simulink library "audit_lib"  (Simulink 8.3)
settings: Solver=ode45  StartTime=0.0  StopTime=10.0  RelTol=1e-3
undefined symbols (not defined in the file or in its folder): convert, VerboseSignal
libraries: audit_lib x23, simulink x16

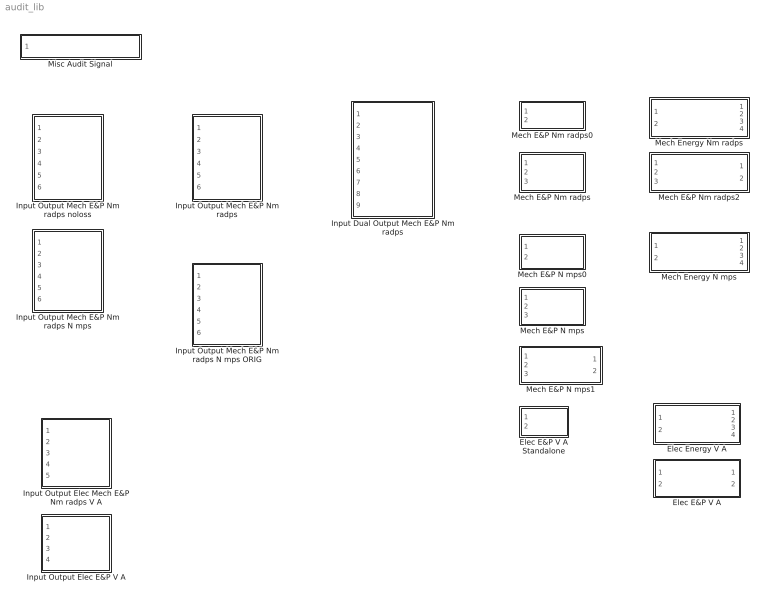
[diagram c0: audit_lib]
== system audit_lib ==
  Elec E&P V A : Subsystem
  Elec E&P V A Standalone : Subsystem
  Elec Energy V A : Subsystem  TreatAsAtomicUnit=on
  Input Dual Output Mech E&P Nm radps : Subsystem
  Input Output Elec E&P V A : Subsystem
  Input Output Elec Mech E&P Nm radps V A : Subsystem
  Input Output Mech E&P Nm radps : Subsystem
  Input Output Mech E&P Nm radps N mps : Subsystem
  Input Output Mech E&P Nm radps N mps ORIG : Subsystem
  Input Output Mech E&P Nm radps noloss : Subsystem
  Mech E&P N mps : Subsystem
  Mech E&P N mps0 : Subsystem
  Mech E&P N mps1 : Subsystem
  Mech E&P Nm radps : Subsystem
  Mech E&P Nm radps0 : Subsystem
  Mech E&P Nm radps2 : Subsystem
  Mech Energy N mps : Subsystem  TreatAsAtomicUnit=on
  Mech Energy Nm radps : Subsystem  TreatAsAtomicUnit=on
  Misc Audit Signal : Subsystem

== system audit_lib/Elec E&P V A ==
  volts_V : Inport
  curr_A : Inport  Port=2
  Compare To Constant : simulink/Logic and Bit Operations/Compare To Constant  relop=>=  const=1  OutDataTypeStr=boolean
  Constant : Constant  Value=VerboseSignal
  Subsystem : Subsystem
  pos_kJ : Outport
  neg_kJ : Outport  Port=2
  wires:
  volts_V/1 -> Subsystem/1(volts_V)
  curr_A/1 -> Subsystem/2(curr_A)
  Subsystem/1(pos_kJ) -> pos_kJ/1
  Subsystem/2(neg_kJ) -> neg_kJ/1
  Compare To Constant/1 -> Subsystem/Enable
  Constant/1 -> Compare To Constant/1

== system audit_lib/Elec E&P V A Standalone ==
  volts_V : Inport
  curr_A : Inport  Port=2
  Compare To Constant : simulink/Logic and Bit Operations/Compare To Constant  relop=>=  const=1  OutDataTypeStr=boolean
  Constant : Constant  Value=VerboseSignal
  Subsystem : Subsystem
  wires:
  volts_V/1 -> Subsystem/1(volts_V)
  curr_A/1 -> Subsystem/2(curr_A)
  Compare To Constant/1 -> Subsystem/Enable
  Constant/1 -> Compare To Constant/1

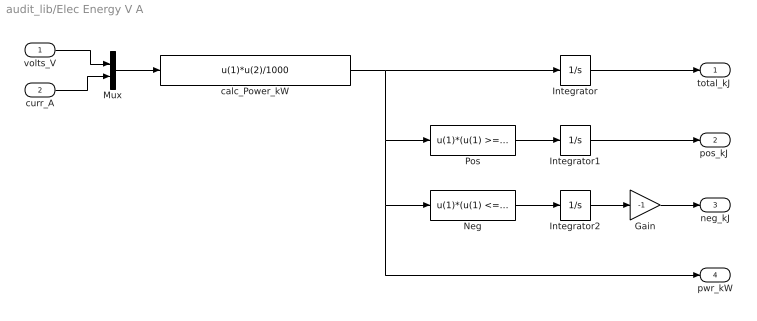
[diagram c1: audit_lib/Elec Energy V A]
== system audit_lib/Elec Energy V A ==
  volts_V : Inport
  curr_A : Inport  Port=2
  Gain : Gain  Gain=-1
  Integrator : Integrator  ZeroCross=off
  Integrator1 : Integrator  ZeroCross=off
  Integrator2 : Integrator  ZeroCross=off
  Mux : Mux  Inputs=2
  Neg : Fcn  Expr=u(1)*(u(1) <= 0)
  Pos : Fcn  Expr=u(1)*(u(1) >= 0)
  calc_Power_kW : Fcn  Expr=u(1)*u(2)/1000
  "total_kJ " : Outport
  "pos_kJ " : Outport  Port=2
  neg_kJ : Outport  Port=3
  pwr_kW : Outport  Port=4
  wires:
  calc_Power_kW/1 -> Pos/1, Neg/1, pwr_kW/1, Integrator/1
  Gain/1 -> neg_kJ/1
  Integrator1/1 -> "pos_kJ "/1
  Integrator2/1 -> Gain/1
  Neg/1 -> Integrator2/1
  Pos/1 -> Integrator1/1
  Integrator/1 -> "total_kJ "/1
  Mux/1 -> calc_Power_kW/1
  volts_V/1 -> Mux/1
  curr_A/1 -> Mux/2

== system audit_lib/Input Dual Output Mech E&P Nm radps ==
  trq_in_Nm : Inport
  spd_in_radps : Inport  Port=2
  iner_in_kgm2 : Inport  Port=3
  trq_out1_Nm : Inport  Port=4
  spd_out1_radps : Inport  Port=5
  iner_out1_kgm2 : Inport  Port=6
  trq_out2_Nm : Inport  Port=7
  spd_out2_radps : Inport  Port=8
  iner_out2_kgm : Inport  Port=9
  Compare To Constant : simulink/Logic and Bit Operations/Compare To Constant  relop=>=  const=1  OutDataTypeStr=boolean
  Constant : Constant  Value=VerboseSignal
  Subsystem : Subsystem
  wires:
  trq_in_Nm/1 -> Subsystem/1(trq_in_Nm)
  spd_in_radps/1 -> Subsystem/2(spd_in_radps)
  iner_in_kgm2/1 -> Subsystem/3(iner_in_kgm2)
  trq_out1_Nm/1 -> Subsystem/4(trq_out1_Nm)
  spd_out1_radps/1 -> Subsystem/5(spd_out1_radps)
  iner_out1_kgm2/1 -> Subsystem/6(iner_out1_kgm2)
  trq_out2_Nm/1 -> Subsystem/7(trq_out2_Nm)
  spd_out2_radps/1 -> Subsystem/8(spd_out2_radps)
  iner_out2_kgm/1 -> Subsystem/9(iner_out2_kgm)
  Compare To Constant/1 -> Subsystem/Enable
  Constant/1 -> Compare To Constant/1

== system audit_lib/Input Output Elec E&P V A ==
  volts_in_V : Inport
  curr_in_A : Inport  Port=2
  volts_out_V : Inport  Port=3
  curr_out_A : Inport  Port=4
  Compare To Constant : simulink/Logic and Bit Operations/Compare To Constant  relop=>=  const=1  OutDataTypeStr=boolean
  Constant : Constant  Value=VerboseSignal
  Subsystem : Subsystem
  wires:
  volts_in_V/1 -> Subsystem/1(volts_in_V)
  curr_in_A/1 -> Subsystem/2(curr_in_A)
  volts_out_V/1 -> Subsystem/3(volts_out_V)
  curr_out_A/1 -> Subsystem/4(curr_out_A)
  Compare To Constant/1 -> Subsystem/Enable
  Constant/1 -> Compare To Constant/1

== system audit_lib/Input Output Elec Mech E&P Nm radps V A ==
  volts_in_V : Inport
  curr_in_A : Inport  Port=2
  trq_out_Nm : Inport  Port=3
  spd_out_radps : Inport  Port=4
  iner_out_kgm2 : Inport  Port=5
  Compare To Constant : simulink/Logic and Bit Operations/Compare To Constant  relop=>=  const=1  OutDataTypeStr=boolean
  Constant : Constant  Value=VerboseSignal
  Subsystem : Subsystem
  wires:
  volts_in_V/1 -> Subsystem/1(volts_in_V)
  curr_in_A/1 -> Subsystem/2(curr_in_A)
  trq_out_Nm/1 -> Subsystem/3(trq_out_Nm)
  spd_out_radps/1 -> Subsystem/4(spd_out_radps)
  iner_out_kgm2/1 -> Subsystem/5(iner_out_kgm2)
  Compare To Constant/1 -> Subsystem/Enable
  Constant/1 -> Compare To Constant/1

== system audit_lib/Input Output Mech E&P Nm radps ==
  trq_in_Nm : Inport
  spd_in_radps : Inport  Port=2
  iner_in_kgm2 : Inport  Port=3
  trq_out_Nm : Inport  Port=4
  spd_out_radps : Inport  Port=5
  iner_out_kgm2 : Inport  Port=6
  Compare To Constant : simulink/Logic and Bit Operations/Compare To Constant  relop=>=  const=1  OutDataTypeStr=boolean
  Constant : Constant  Value=VerboseSignal
  Subsystem : Subsystem
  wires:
  trq_in_Nm/1 -> Subsystem/1(trq_in_Nm)
  spd_in_radps/1 -> Subsystem/2(spd_in_radps)
  iner_in_kgm2/1 -> Subsystem/3(iner_in_kgm2)
  trq_out_Nm/1 -> Subsystem/4(trq_out_Nm)
  spd_out_radps/1 -> Subsystem/5(spd_out_radps)
  iner_out_kgm2/1 -> Subsystem/6(iner_out_kgm2)
  Compare To Constant/1 -> Subsystem/Enable
  Constant/1 -> Compare To Constant/1

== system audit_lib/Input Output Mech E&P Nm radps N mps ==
  trq_in_Nm : Inport
  spd_in_radps : Inport  Port=2
  iner_in_kgm2 : Inport  Port=3
  frc_out_N : Inport  Port=4
  spd_out_mps : Inport  Port=5
  mass_out_kg : Inport  Port=6
  Compare To Constant : simulink/Logic and Bit Operations/Compare To Constant  relop=>=  const=1  OutDataTypeStr=boolean
  Constant : Constant  Value=VerboseSignal
  Subsystem : Subsystem
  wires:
  trq_in_Nm/1 -> Subsystem/1(trq_in_Nm)
  spd_in_radps/1 -> Subsystem/2(spd_in_radps)
  iner_in_kgm2/1 -> Subsystem/3(iner_in_kgm2)
  frc_out_N/1 -> Subsystem/4(frc_out_N)
  spd_out_mps/1 -> Subsystem/5(spd_out_mps)
  mass_out_kg/1 -> Subsystem/6(mass_out_kg)
  Compare To Constant/1 -> Subsystem/Enable
  Constant/1 -> Compare To Constant/1

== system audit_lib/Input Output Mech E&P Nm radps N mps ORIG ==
  trq_in_Nm : Inport
  spd_in_radps : Inport  Port=2
  iner_in_kgm2 : Inport  Port=3
  frc_out_N : Inport  Port=4
  spd_out_mps : Inport  Port=5
  mass_out_kg : Inport  Port=6
  Compare To Constant : simulink/Logic and Bit Operations/Compare To Constant  relop=>=  const=1  OutDataTypeStr=boolean
  Constant : Constant  Value=VerboseSignal
  Subsystem : Subsystem
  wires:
  Constant/1 -> Compare To Constant/1
  Compare To Constant/1 -> Subsystem/Enable
  mass_out_kg/1 -> Subsystem/6(mass_out_kg)
  spd_out_mps/1 -> Subsystem/5(spd_out_mps)
  frc_out_N/1 -> Subsystem/4(frc_out_N)
  iner_in_kgm2/1 -> Subsystem/3(iner_in_kgm2)
  spd_in_radps/1 -> Subsystem/2(spd_in_radps)
  trq_in_Nm/1 -> Subsystem/1(trq_in_Nm)

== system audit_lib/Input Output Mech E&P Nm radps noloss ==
  trq_in_Nm : Inport
  spd_in_radps : Inport  Port=2
  iner_in_kgm2 : Inport  Port=3
  trq_out_Nm : Inport  Port=4
  spd_out_radps : Inport  Port=5
  iner_out_kgm2 : Inport  Port=6
  Compare To Constant : simulink/Logic and Bit Operations/Compare To Constant  relop=>=  const=1  OutDataTypeStr=boolean
  Constant : Constant  Value=VerboseSignal
  Subsystem : Subsystem
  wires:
  trq_in_Nm/1 -> Subsystem/1(trq_in_Nm)
  spd_in_radps/1 -> Subsystem/2(spd_in_radps)
  iner_in_kgm2/1 -> Subsystem/3(iner_in_kgm2)
  trq_out_Nm/1 -> Subsystem/4(trq_out_Nm)
  spd_out_radps/1 -> Subsystem/5(spd_out_radps)
  iner_out_kgm2/1 -> Subsystem/6(iner_out_kgm2)
  Compare To Constant/1 -> Subsystem/Enable
  Constant/1 -> Compare To Constant/1

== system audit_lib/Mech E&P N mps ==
  force_N : Inport
  spd_mps : Inport  Port=2
  mass_kg : Inport  Port=3
  Compare To Constant : simulink/Logic and Bit Operations/Compare To Constant  relop=>=  const=1  OutDataTypeStr=boolean
  Constant : Constant  Value=VerboseSignal
  Subsystem : Subsystem
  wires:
  force_N/1 -> Subsystem/1(force_N)
  spd_mps/1 -> Subsystem/2(spd_mps)
  mass_kg/1 -> Subsystem/3(mass_kg)
  Compare To Constant/1 -> Subsystem/Enable
  Constant/1 -> Compare To Constant/1

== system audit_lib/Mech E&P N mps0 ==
  force_N : Inport
  spd_mps : Inport  Port=2
  Compare To Constant : simulink/Logic and Bit Operations/Compare To Constant  relop=>=  const=1  OutDataTypeStr=boolean
  Constant : Constant  Value=VerboseSignal
  Subsystem : Subsystem
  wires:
  force_N/1 -> Subsystem/1(force_N)
  spd_mps/1 -> Subsystem/2(spd_mps)
  Compare To Constant/1 -> Subsystem/Enable
  Constant/1 -> Compare To Constant/1

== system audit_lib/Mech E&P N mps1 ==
  force_N : Inport
  spd_mps : Inport  Port=2
  mass_kg : Inport  Port=3
  Compare To Constant : simulink/Logic and Bit Operations/Compare To Constant  relop=>=  const=1  OutDataTypeStr=boolean
  Constant : Constant  Value=VerboseSignal
  Subsystem : Subsystem
  pos_kJ : Outport
  neg_kJ : Outport  Port=2
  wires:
  Constant/1 -> Compare To Constant/1
  Compare To Constant/1 -> Subsystem/Enable
  mass_kg/1 -> Subsystem/3(mass_kg)
  spd_mps/1 -> Subsystem/2(spd_mps)
  force_N/1 -> Subsystem/1(force_N)
  Subsystem/1(pos_kJ) -> pos_kJ/1
  Subsystem/2(neg_kJ) -> neg_kJ/1

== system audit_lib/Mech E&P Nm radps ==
  " trq_Nm" : Inport
  spd_radps : Inport  Port=2
  iner_kgm2 : Inport  Port=3
  Compare To Constant : simulink/Logic and Bit Operations/Compare To Constant  relop=>=  const=1  OutDataTypeStr=boolean
  Constant : Constant  Value=VerboseSignal
  Subsystem : Subsystem
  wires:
  " trq_Nm"/1 -> Subsystem/1(" trq_Nm")
  spd_radps/1 -> Subsystem/2(spd_radps)
  iner_kgm2/1 -> Subsystem/3(iner_kgm2)
  Compare To Constant/1 -> Subsystem/Enable
  Constant/1 -> Compare To Constant/1

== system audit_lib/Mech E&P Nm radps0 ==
  trq_Nm : Inport
  spd_radps : Inport  Port=2
  Compare To Constant : simulink/Logic and Bit Operations/Compare To Constant  relop=>=  const=1  OutDataTypeStr=boolean
  Constant : Constant  Value=VerboseSignal
  Subsystem : Subsystem
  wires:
  trq_Nm/1 -> Subsystem/1(trq_Nm)
  spd_radps/1 -> Subsystem/2(spd_radps)
  Compare To Constant/1 -> Subsystem/Enable
  Constant/1 -> Compare To Constant/1

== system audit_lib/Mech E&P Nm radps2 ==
  " trq_Nm" : Inport
  spd_radps : Inport  Port=2
  iner_kgm2 : Inport  Port=3
  Compare To Constant : simulink/Logic and Bit Operations/Compare To Constant  relop=>=  const=1  OutDataTypeStr=boolean
  Constant : Constant  Value=VerboseSignal
  Subsystem : Subsystem
  pos_kJ : Outport
  neg_kJ : Outport  Port=2
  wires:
  " trq_Nm"/1 -> Subsystem/1(" trq_Nm")
  spd_radps/1 -> Subsystem/2(spd_radps)
  iner_kgm2/1 -> Subsystem/3(iner_kgm2)
  Compare To Constant/1 -> Subsystem/Enable
  Subsystem/1(pos_kJ) -> pos_kJ/1
  Subsystem/2(neg_kJ) -> neg_kJ/1
  Constant/1 -> Compare To Constant/1

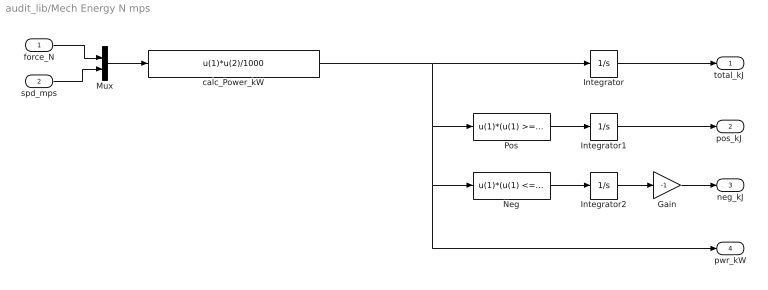
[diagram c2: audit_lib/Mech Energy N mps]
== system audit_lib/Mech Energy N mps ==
  force_N : Inport
  spd_mps : Inport  Port=2
  Gain : Gain  Gain=-1
  Integrator : Integrator  ZeroCross=off
  Integrator1 : Integrator  ZeroCross=off
  Integrator2 : Integrator  ZeroCross=off
  Mux : Mux  Inputs=2
  Neg : Fcn  Expr=u(1)*(u(1) <= 0)
  Pos : Fcn  Expr=u(1)*(u(1) >= 0)
  calc_Power_kW : Fcn  Expr=u(1)*u(2)/1000
  "total_kJ " : Outport
  "pos_kJ " : Outport  Port=2
  neg_kJ : Outport  Port=3
  pwr_kW : Outport  Port=4
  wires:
  spd_mps/1 -> Mux/2
  force_N/1 -> Mux/1
  Mux/1 -> calc_Power_kW/1
  Integrator/1 -> "total_kJ "/1
  Pos/1 -> Integrator1/1
  Neg/1 -> Integrator2/1
  Integrator2/1 -> Gain/1
  Integrator1/1 -> "pos_kJ "/1
  Gain/1 -> neg_kJ/1
  calc_Power_kW/1 -> Integrator/1, pwr_kW/1, Neg/1, Pos/1

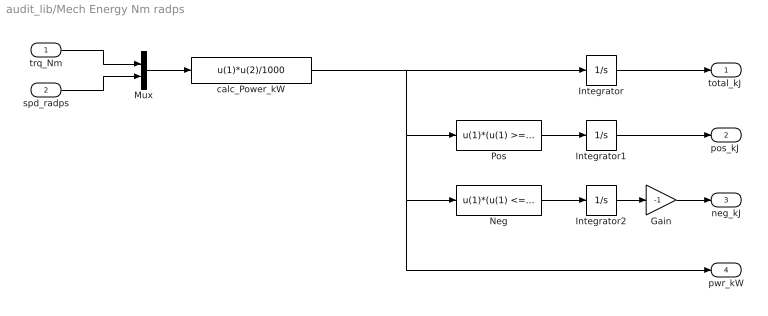
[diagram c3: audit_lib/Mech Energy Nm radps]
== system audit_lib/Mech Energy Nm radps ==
  trq_Nm : Inport
  spd_radps : Inport  Port=2
  Gain : Gain  Gain=-1
  Integrator : Integrator  ZeroCross=off
  Integrator1 : Integrator  ZeroCross=off
  Integrator2 : Integrator  ZeroCross=off
  Mux : Mux  Inputs=2
  Neg : Fcn  Expr=u(1)*(u(1) <= 0)
  Pos : Fcn  Expr=u(1)*(u(1) >= 0)
  calc_Power_kW : Fcn  Expr=u(1)*u(2)/1000
  "total_kJ " : Outport
  "pos_kJ " : Outport  Port=2
  neg_kJ : Outport  Port=3
  pwr_kW : Outport  Port=4
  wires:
  Integrator/1 -> "total_kJ "/1
  Mux/1 -> calc_Power_kW/1
  trq_Nm/1 -> Mux/1
  spd_radps/1 -> Mux/2
  Pos/1 -> Integrator1/1
  Neg/1 -> Integrator2/1
  Integrator2/1 -> Gain/1
  Integrator1/1 -> "pos_kJ "/1
  Gain/1 -> neg_kJ/1
  calc_Power_kW/1 -> Integrator/1, pwr_kW/1, Neg/1, Pos/1

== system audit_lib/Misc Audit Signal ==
  Var : Inport
  Compare To Constant : simulink/Logic and Bit Operations/Compare To Constant  relop=>=  const=1  OutDataTypeStr=boolean
  Constant : Constant  Value=VerboseSignal
  Subsystem : Subsystem
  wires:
  Var/1 -> Subsystem/1(In1)
  Compare To Constant/1 -> Subsystem/Enable
  Constant/1 -> Compare To Constant/1

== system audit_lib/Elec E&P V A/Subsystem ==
  volts_V : Inport
  curr_A : Inport  Port=2
  Enable : EnablePort  ZeroCross=off
  Elec Energy V A : audit_lib/Elec Energy V A
  amps_to_workspace : ToWorkspace  VariableName=audit__elec__emachine_Amps  SampleTime=-1
  energy_to_workspace : ToWorkspace  VariableName=audit__elec__emachine_kJ  SampleTime=-1
  neg_energy_to_workspace : ToWorkspace  VariableName=audit__elec__emachine_neg_kJ  SampleTime=-1
  pos_energy_to_workspace : ToWorkspace  VariableName=audit__elec__emachine_pos_kJ  SampleTime=-1
  power_to_workspace : ToWorkspace  VariableName=audit__elec__emachine_kW  SampleTime=-1
  volts_to_workspace : ToWorkspace  VariableName=audit__elec__emachine_Volts  SampleTime=-1
  pos_kJ : Outport  InitialOutput=0
  neg_kJ : Outport  Port=2  InitialOutput=0
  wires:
  Elec Energy V A/3 -> neg_kJ/1, neg_energy_to_workspace/1
  Elec Energy V A/4 -> power_to_workspace/1
  Elec Energy V A/2 -> pos_kJ/1, pos_energy_to_workspace/1
  Elec Energy V A/1 -> energy_to_workspace/1
  volts_V/1 -> volts_to_workspace/1, Elec Energy V A/1
  curr_A/1 -> amps_to_workspace/1, Elec Energy V A/2

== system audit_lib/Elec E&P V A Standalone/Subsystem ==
  volts_V : Inport
  curr_A : Inport  Port=2
  Enable : EnablePort  ZeroCross=off
  Elec Energy V A : audit_lib/Elec Energy V A
  amps_to_workspace : ToWorkspace  VariableName=audit__elec__emachine_Amps  SampleTime=-1
  energy_to_workspace : ToWorkspace  VariableName=audit__elec__emachine_kJ  SampleTime=-1
  neg_energy_to_workspace : ToWorkspace  VariableName=audit__elec__emachine_neg_kJ  SampleTime=-1
  pos_energy_to_workspace : ToWorkspace  VariableName=audit__elec__emachine_pos_kJ  SampleTime=-1
  power_to_workspace : ToWorkspace  VariableName=audit__elec__emachine_kW  SampleTime=-1
  volts_to_workspace : ToWorkspace  VariableName=audit__elec__emachine_Volts  SampleTime=-1
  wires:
  volts_V/1 -> Elec Energy V A/1, volts_to_workspace/1
  curr_A/1 -> Elec Energy V A/2, amps_to_workspace/1
  Elec Energy V A/3 -> neg_energy_to_workspace/1
  Elec Energy V A/2 -> pos_energy_to_workspace/1
  Elec Energy V A/4 -> power_to_workspace/1
  Elec Energy V A/1 -> energy_to_workspace/1

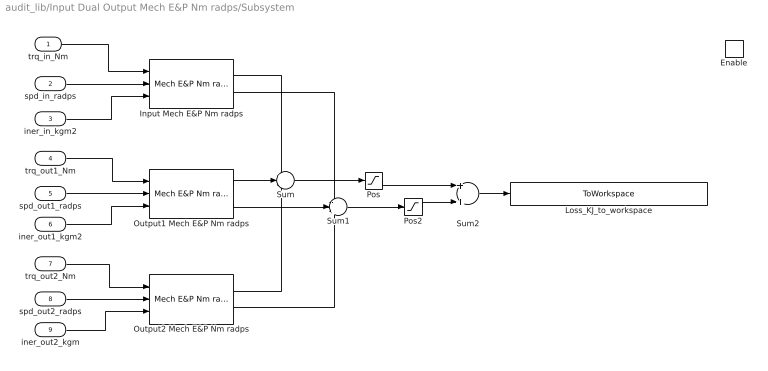
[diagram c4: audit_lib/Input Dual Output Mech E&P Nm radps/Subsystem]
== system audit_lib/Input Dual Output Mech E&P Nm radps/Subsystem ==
  trq_in_Nm : Inport
  spd_in_radps : Inport  Port=2
  iner_in_kgm2 : Inport  Port=3
  trq_out1_Nm : Inport  Port=4
  spd_out1_radps : Inport  Port=5
  iner_out1_kgm2 : Inport  Port=6
  trq_out2_Nm : Inport  Port=7
  spd_out2_radps : Inport  Port=8
  iner_out2_kgm : Inport  Port=9
  Enable : EnablePort  ZeroCross=off
  Input Mech E&P Nm radps : audit_lib/Mech E&P Nm radps2  base_name=clutch__input  VerboseSignal=REVS.verbose
  Loss_KJ_to_workspace : ToWorkspace  VariableName=audit__mech__clutch__loss_kJ  SampleTime=-1
  Output1 Mech E&P Nm radps : audit_lib/Mech E&P Nm radps2  base_name=clutch__output1  VerboseSignal=REVS.verbose
  Output2 Mech E&P Nm radps : audit_lib/Mech E&P Nm radps2  base_name=clutch__output2  VerboseSignal=REVS.verbose
  Pos : Saturate  UpperLimit=Inf  LowerLimit=0  ZeroCross=off
  Pos2 : Saturate  UpperLimit=Inf  LowerLimit=0  ZeroCross=off
  Sum : Sum  Inputs=+--
  Sum1 : Sum  Inputs=-++
  Sum2 : Sum
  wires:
  Output2 Mech E&P Nm radps/1 -> Sum/3
  Output2 Mech E&P Nm radps/2 -> Sum1/3
  iner_out2_kgm/1 -> Output2 Mech E&P Nm radps/3
  spd_out2_radps/1 -> Output2 Mech E&P Nm radps/2
  trq_out2_Nm/1 -> Output2 Mech E&P Nm radps/1
  Pos2/1 -> Sum2/2
  Pos/1 -> Sum2/1
  trq_in_Nm/1 -> Input Mech E&P Nm radps/1
  spd_in_radps/1 -> Input Mech E&P Nm radps/2
  trq_out1_Nm/1 -> Output1 Mech E&P Nm radps/1
  spd_out1_radps/1 -> Output1 Mech E&P Nm radps/2
  iner_in_kgm2/1 -> Input Mech E&P Nm radps/3
  iner_out1_kgm2/1 -> Output1 Mech E&P Nm radps/3
  Input Mech E&P Nm radps/1 -> Sum/1
  Output1 Mech E&P Nm radps/1 -> Sum/2
  Output1 Mech E&P Nm radps/2 -> Sum1/2
  Input Mech E&P Nm radps/2 -> Sum1/1
  Sum/1 -> Pos/1
  Sum1/1 -> Pos2/1
  Sum2/1 -> Loss_KJ_to_workspace/1

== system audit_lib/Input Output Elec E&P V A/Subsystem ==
  volts_in_V : Inport
  curr_in_A : Inport  Port=2
  volts_out_V : Inport  Port=3
  curr_out_A : Inport  Port=4
  Enable : EnablePort
  Input Elec E&P V A : audit_lib/Elec E&P V A  base_name=econverter__input  VerboseSignal=REVS.verbose
  Loss_KJ_to_workspace : ToWorkspace  VariableName=audit__elec__econverter__loss_kJ  SampleTime=-1
  Output Elec E&P V A : audit_lib/Elec E&P V A  base_name=econverter__output  VerboseSignal=REVS.verbose
  Pos : Saturate  UpperLimit=Inf  LowerLimit=0  ZeroCross=off
  Pos2 : Saturate  UpperLimit=Inf  LowerLimit=0  ZeroCross=off
  Sum : Sum  Inputs=+-|
  Sum1 : Sum  Inputs=|-+
  Sum2 : Sum
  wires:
  Input Elec E&P V A/1 -> Sum/1
  Sum2/1 -> Loss_KJ_to_workspace/1
  Sum1/1 -> Pos2/1
  Sum/1 -> Pos/1
  Output Elec E&P V A/2 -> Sum1/2
  Input Elec E&P V A/2 -> Sum1/1
  Output Elec E&P V A/1 -> Sum/2
  curr_in_A/1 -> Input Elec E&P V A/2
  volts_in_V/1 -> Input Elec E&P V A/1
  Pos/1 -> Sum2/2
  Pos2/1 -> Sum2/1
  curr_out_A/1 -> Output Elec E&P V A/2
  volts_out_V/1 -> Output Elec E&P V A/1

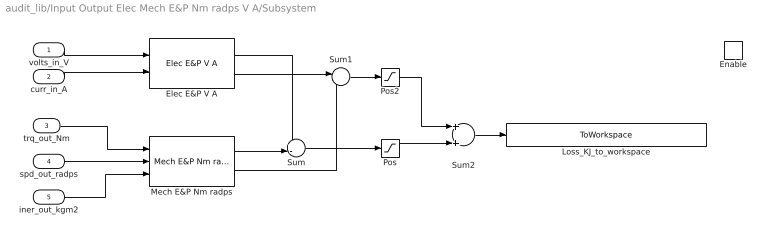
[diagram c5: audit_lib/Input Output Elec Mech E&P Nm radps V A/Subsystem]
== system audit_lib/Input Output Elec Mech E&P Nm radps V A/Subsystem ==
  volts_in_V : Inport
  curr_in_A : Inport  Port=2
  trq_out_Nm : Inport  Port=3
  spd_out_radps : Inport  Port=4
  iner_out_kgm2 : Inport  Port=5
  Enable : EnablePort
  Elec E&P V A : audit_lib/Elec E&P V A  base_name=emachine__input  VerboseSignal=REVS.verbose
  Loss_KJ_to_workspace : ToWorkspace  VariableName=audit__mech__emachine__loss_kJ  SampleTime=-1
  Mech E&P Nm radps : audit_lib/Mech E&P Nm radps2  base_name=emachine__output  VerboseSignal=REVS.verbose
  Pos : Saturate  UpperLimit=Inf  LowerLimit=0  ZeroCross=off
  Pos2 : Saturate  UpperLimit=Inf  LowerLimit=0  ZeroCross=off
  Sum : Sum  Inputs=+-|
  Sum1 : Sum  Inputs=|-+
  Sum2 : Sum
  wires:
  Pos2/1 -> Sum2/1
  Pos/1 -> Sum2/2
  trq_out_Nm/1 -> Mech E&P Nm radps/1
  spd_out_radps/1 -> Mech E&P Nm radps/2
  volts_in_V/1 -> Elec E&P V A/1
  curr_in_A/1 -> Elec E&P V A/2
  iner_out_kgm2/1 -> Mech E&P Nm radps/3
  Mech E&P Nm radps/1 -> Sum/2
  Elec E&P V A/2 -> Sum1/1
  Mech E&P Nm radps/2 -> Sum1/2
  Sum/1 -> Pos/1
  Sum1/1 -> Pos2/1
  Sum2/1 -> Loss_KJ_to_workspace/1
  Elec E&P V A/1 -> Sum/1

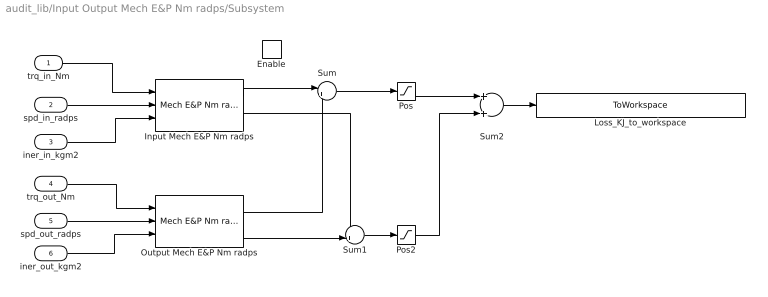
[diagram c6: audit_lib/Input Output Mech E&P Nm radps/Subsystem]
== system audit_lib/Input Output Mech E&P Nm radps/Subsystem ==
  trq_in_Nm : Inport
  spd_in_radps : Inport  Port=2
  iner_in_kgm2 : Inport  Port=3
  trq_out_Nm : Inport  Port=4
  spd_out_radps : Inport  Port=5
  iner_out_kgm2 : Inport  Port=6
  Enable : EnablePort  ZeroCross=off
  Input Mech E&P Nm radps : audit_lib/Mech E&P Nm radps2  base_name=torque_converter__input  VerboseSignal=REVS.verbose
  Loss_KJ_to_workspace : ToWorkspace  VariableName=audit__mech__torque_converter__loss_kJ  SampleTime=-1
  Output Mech E&P Nm radps : audit_lib/Mech E&P Nm radps2  base_name=torque_converter__output  VerboseSignal=REVS.verbose
  Pos : Saturate  UpperLimit=Inf  LowerLimit=0  ZeroCross=off
  Pos2 : Saturate  UpperLimit=Inf  LowerLimit=0  ZeroCross=off
  Sum : Sum  Inputs=|+-
  Sum1 : Sum  Inputs=-+|
  Sum2 : Sum
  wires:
  Pos2/1 -> Sum2/2
  Pos/1 -> Sum2/1
  trq_in_Nm/1 -> Input Mech E&P Nm radps/1
  spd_in_radps/1 -> Input Mech E&P Nm radps/2
  trq_out_Nm/1 -> Output Mech E&P Nm radps/1
  spd_out_radps/1 -> Output Mech E&P Nm radps/2
  iner_in_kgm2/1 -> Input Mech E&P Nm radps/3
  iner_out_kgm2/1 -> Output Mech E&P Nm radps/3
  Input Mech E&P Nm radps/1 -> Sum/1
  Output Mech E&P Nm radps/1 -> Sum/2
  Output Mech E&P Nm radps/2 -> Sum1/2
  Input Mech E&P Nm radps/2 -> Sum1/1
  Sum/1 -> Pos/1
  Sum1/1 -> Pos2/1
  Sum2/1 -> Loss_KJ_to_workspace/1

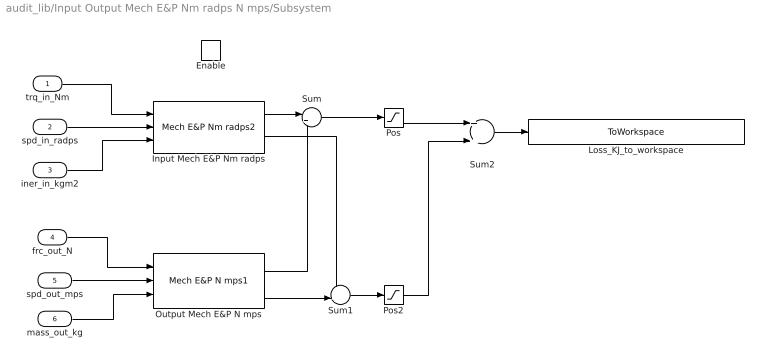
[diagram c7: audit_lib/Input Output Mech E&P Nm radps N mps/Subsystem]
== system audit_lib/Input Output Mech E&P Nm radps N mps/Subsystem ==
  trq_in_Nm : Inport
  spd_in_radps : Inport  Port=2
  iner_in_kgm2 : Inport  Port=3
  frc_out_N : Inport  Port=4
  spd_out_mps : Inport  Port=5
  mass_out_kg : Inport  Port=6
  Enable : EnablePort  ZeroCross=off
  Input Mech E&P Nm radps : audit_lib/Mech E&P Nm radps2  base_name=device__input  VerboseSignal=REVS.verbose
  Loss_KJ_to_workspace : ToWorkspace  VariableName=audit__mech__device__loss_kJ  SampleTime=-1
  Output Mech E&P N mps : audit_lib/Mech E&P N mps1  base_name=device__output  VerboseSignal=REVS.verbose
  Pos : Saturate  UpperLimit=Inf  LowerLimit=0  ZeroCross=off
  Pos2 : Saturate  UpperLimit=Inf  LowerLimit=0  ZeroCross=off
  Sum : Sum  Inputs=|+-
  Sum1 : Sum  Inputs=-+|
  Sum2 : Sum
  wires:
  spd_out_mps/1 -> Output Mech E&P N mps/2
  frc_out_N/1 -> Output Mech E&P N mps/1
  spd_in_radps/1 -> Input Mech E&P Nm radps/2
  trq_in_Nm/1 -> Input Mech E&P Nm radps/1
  iner_in_kgm2/1 -> Input Mech E&P Nm radps/3
  mass_out_kg/1 -> Output Mech E&P N mps/3
  Pos2/1 -> Sum2/2
  Pos/1 -> Sum2/1
  Input Mech E&P Nm radps/1 -> Sum/1
  Output Mech E&P N mps/1 -> Sum/2
  Output Mech E&P N mps/2 -> Sum1/2
  Input Mech E&P Nm radps/2 -> Sum1/1
  Sum/1 -> Pos/1
  Sum1/1 -> Pos2/1
  Sum2/1 -> Loss_KJ_to_workspace/1

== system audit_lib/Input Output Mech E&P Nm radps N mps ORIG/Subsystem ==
  trq_in_Nm : Inport
  spd_in_radps : Inport  Port=2
  iner_in_kgm2 : Inport  Port=3
  frc_out_N : Inport  Port=4
  spd_out_mps : Inport  Port=5
  mass_out_kg : Inport  Port=6
  Enable : EnablePort  ZeroCross=off
  Input Mech E&P Nm radps : audit_lib/Mech E&P Nm radps  base_name=device__input  VerboseSignal=REVS.verbose
  Output Mech E&P N mps : audit_lib/Mech E&P N mps  base_name=device__output  VerboseSignal=REVS.verbose
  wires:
  mass_out_kg/1 -> Output Mech E&P N mps/3
  iner_in_kgm2/1 -> Input Mech E&P Nm radps/3
  trq_in_Nm/1 -> Input Mech E&P Nm radps/1
  spd_in_radps/1 -> Input Mech E&P Nm radps/2
  frc_out_N/1 -> Output Mech E&P N mps/1
  spd_out_mps/1 -> Output Mech E&P N mps/2

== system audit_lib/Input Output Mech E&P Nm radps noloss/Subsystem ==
  trq_in_Nm : Inport
  spd_in_radps : Inport  Port=2
  iner_in_kgm2 : Inport  Port=3
  trq_out_Nm : Inport  Port=4
  spd_out_radps : Inport  Port=5
  iner_out_kgm2 : Inport  Port=6
  Enable : EnablePort  ZeroCross=off
  Input Mech E&P Nm radps : audit_lib/Mech E&P Nm radps  base_name=device__input  VerboseSignal=REVS.verbose
  Output Mech E&P Nm radps : audit_lib/Mech E&P Nm radps  base_name=device__output  VerboseSignal=REVS.verbose
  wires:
  spd_in_radps/1 -> Input Mech E&P Nm radps/2
  spd_out_radps/1 -> Output Mech E&P Nm radps/2
  iner_out_kgm2/1 -> Output Mech E&P Nm radps/3
  trq_in_Nm/1 -> Input Mech E&P Nm radps/1
  trq_out_Nm/1 -> Output Mech E&P Nm radps/1
  iner_in_kgm2/1 -> Input Mech E&P Nm radps/3

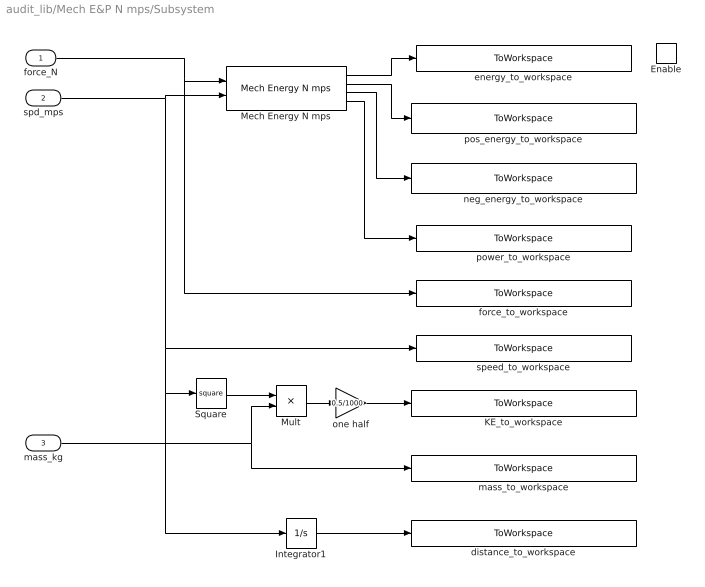
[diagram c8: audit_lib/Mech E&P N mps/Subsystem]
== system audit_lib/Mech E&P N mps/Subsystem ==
  force_N : Inport
  spd_mps : Inport  Port=2
  mass_kg : Inport  Port=3
  Enable : EnablePort  ZeroCross=off
  Integrator1 : Integrator  LimitOutput=on  UpperSaturationLimit=Inf  LowerSaturationLimit=0  ZeroCross=off
  KE_to_workspace : ToWorkspace  VariableName=audit__mech__device_KE_kJ  SampleTime=-1
  Mech Energy N mps : audit_lib/Mech Energy N mps
  Mult : Product  Inputs=**
  Square : Math  Operator=square
  distance_to_workspace : ToWorkspace  VariableName=audit__mech__device_m  SampleTime=-1
  energy_to_workspace : ToWorkspace  VariableName=audit__mech__device_kJ  SampleTime=-1
  force_to_workspace : ToWorkspace  VariableName=audit__mech__device_N  SampleTime=-1
  mass_to_workspace : ToWorkspace  VariableName=audit__mech__device_kg  SampleTime=-1
  neg_energy_to_workspace : ToWorkspace  VariableName=audit__mech__device_neg_kJ  SampleTime=-1
  one half : Gain  Gain=0.5/1000
  pos_energy_to_workspace : ToWorkspace  VariableName=audit__mech__device_pos_kJ  SampleTime=-1
  power_to_workspace : ToWorkspace  VariableName=audit__mech__device_kW  SampleTime=-1
  speed_to_workspace : ToWorkspace  VariableName=audit__mech__device_mps  SampleTime=-1
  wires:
  Mech Energy N mps/1 -> energy_to_workspace/1
  Mech Energy N mps/4 -> power_to_workspace/1
  Mech Energy N mps/2 -> pos_energy_to_workspace/1
  Mech Energy N mps/3 -> neg_energy_to_workspace/1
  one half/1 -> KE_to_workspace/1
  Square/1 -> Mult/1
  Mult/1 -> one half/1
  mass_kg/1 -> Mult/2, mass_to_workspace/1
  spd_mps/1 -> Mech Energy N mps/2, Integrator1/1, Square/1, speed_to_workspace/1
  force_N/1 -> Mech Energy N mps/1, force_to_workspace/1
  Integrator1/1 -> distance_to_workspace/1

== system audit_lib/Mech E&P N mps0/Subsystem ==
  force_N : Inport
  spd_mps : Inport  Port=2
  Enable : EnablePort  ZeroCross=off
  Integrator1 : Integrator  LimitOutput=on  UpperSaturationLimit=Inf  LowerSaturationLimit=0  ZeroCross=off
  Mech Energy N mps : audit_lib/Mech Energy N mps
  distance_to_workspace : ToWorkspace  VariableName=audit__mech__device_m  SampleTime=-1
  energy_to_workspace : ToWorkspace  VariableName=audit__mech__device_kJ  SampleTime=-1
  force_to_workspace : ToWorkspace  VariableName=audit__mech__device_N  SampleTime=-1
  neg_energy_to_workspace : ToWorkspace  VariableName=audit__mech__device_neg_kJ  SampleTime=-1
  pos_energy_to_workspace : ToWorkspace  VariableName=audit__mech__device_pos_kJ  SampleTime=-1
  power_to_workspace : ToWorkspace  VariableName=audit__mech__device_kW  SampleTime=-1
  speed_to_workspace : ToWorkspace  VariableName=audit__mech__device_mps  SampleTime=-1
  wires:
  Mech Energy N mps/3 -> neg_energy_to_workspace/1
  Mech Energy N mps/2 -> pos_energy_to_workspace/1
  Mech Energy N mps/4 -> power_to_workspace/1
  Mech Energy N mps/1 -> energy_to_workspace/1
  force_N/1 -> force_to_workspace/1, Mech Energy N mps/1
  spd_mps/1 -> Integrator1/1, speed_to_workspace/1, Mech Energy N mps/2
  Integrator1/1 -> distance_to_workspace/1

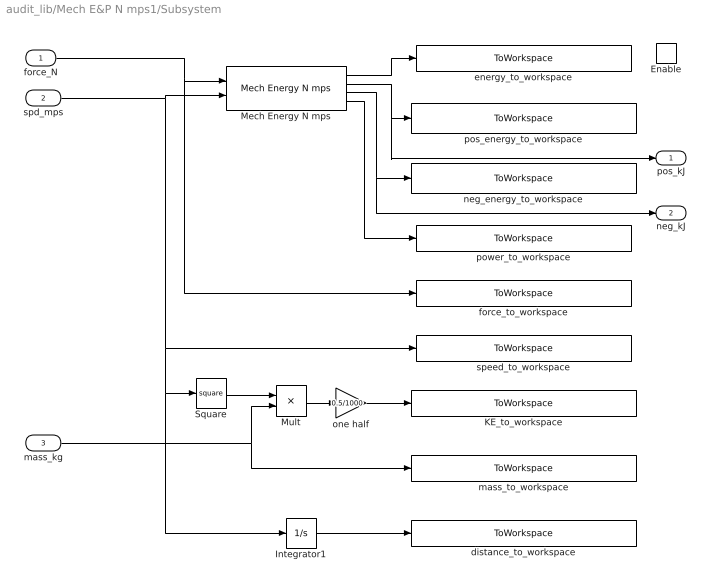
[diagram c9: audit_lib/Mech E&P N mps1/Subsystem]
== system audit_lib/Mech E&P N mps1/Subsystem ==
  force_N : Inport
  spd_mps : Inport  Port=2
  mass_kg : Inport  Port=3
  Enable : EnablePort  ZeroCross=off
  Integrator1 : Integrator  LimitOutput=on  UpperSaturationLimit=Inf  LowerSaturationLimit=0  ZeroCross=off
  KE_to_workspace : ToWorkspace  VariableName=audit__mech__device_KE_kJ  SampleTime=-1
  Mech Energy N mps : audit_lib/Mech Energy N mps
  Mult : Product  Inputs=**
  Square : Math  Operator=square
  distance_to_workspace : ToWorkspace  VariableName=audit__mech__device_m  SampleTime=-1
  energy_to_workspace : ToWorkspace  VariableName=audit__mech__device_kJ  SampleTime=-1
  force_to_workspace : ToWorkspace  VariableName=audit__mech__device_N  SampleTime=-1
  mass_to_workspace : ToWorkspace  VariableName=audit__mech__device_kg  SampleTime=-1
  neg_energy_to_workspace : ToWorkspace  VariableName=audit__mech__device_neg_kJ  SampleTime=-1
  one half : Gain  Gain=0.5/1000
  pos_energy_to_workspace : ToWorkspace  VariableName=audit__mech__device_pos_kJ  SampleTime=-1
  power_to_workspace : ToWorkspace  VariableName=audit__mech__device_kW  SampleTime=-1
  speed_to_workspace : ToWorkspace  VariableName=audit__mech__device_mps  SampleTime=-1
  pos_kJ : Outport
  neg_kJ : Outport  Port=2
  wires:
  Integrator1/1 -> distance_to_workspace/1
  force_N/1 -> force_to_workspace/1, Mech Energy N mps/1
  spd_mps/1 -> speed_to_workspace/1, Square/1, Integrator1/1, Mech Energy N mps/2
  mass_kg/1 -> mass_to_workspace/1, Mult/2
  Mult/1 -> one half/1
  Square/1 -> Mult/1
  one half/1 -> KE_to_workspace/1
  Mech Energy N mps/4 -> power_to_workspace/1
  Mech Energy N mps/1 -> energy_to_workspace/1
  Mech Energy N mps/2 -> pos_kJ/1, pos_energy_to_workspace/1
  Mech Energy N mps/3 -> neg_kJ/1, neg_energy_to_workspace/1

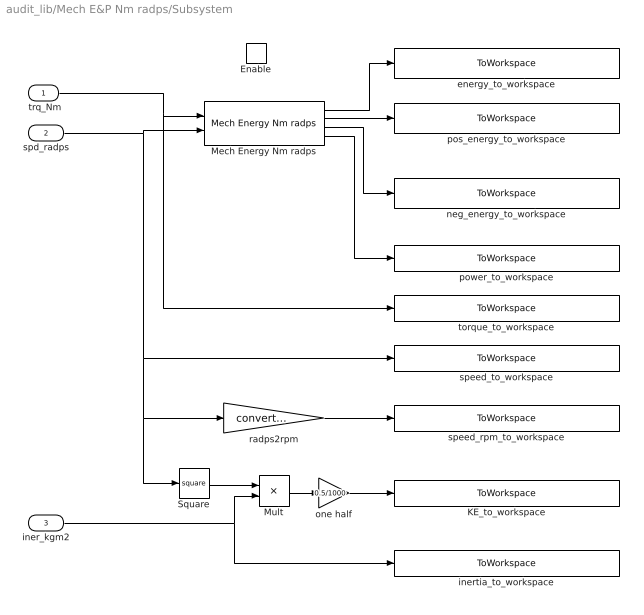
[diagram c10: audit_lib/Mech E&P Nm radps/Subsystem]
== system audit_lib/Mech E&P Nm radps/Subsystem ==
  " trq_Nm" : Inport
  spd_radps : Inport  Port=2
  iner_kgm2 : Inport  Port=3
  Enable : EnablePort  ZeroCross=off
  KE_to_workspace : ToWorkspace  VariableName=audit__mech__device_KE_kJ  SampleTime=-1
  Mech Energy Nm radps : audit_lib/Mech Energy Nm radps
  Mult : Product  Inputs=**
  Square : Math  Operator=square
  energy_to_workspace : ToWorkspace  VariableName=audit__mech__device_kJ  SampleTime=-1
  inertia_to_workspace : ToWorkspace  VariableName=audit__mech__device_kgm2  SampleTime=-1
  neg_energy_to_workspace : ToWorkspace  VariableName=audit__mech__device_neg_kJ  SampleTime=-1
  one half : Gain  Gain=0.5/1000
  pos_energy_to_workspace : ToWorkspace  VariableName=audit__mech__device_pos_kJ  SampleTime=-1
  power_to_workspace : ToWorkspace  VariableName=audit__mech__device_kW  SampleTime=-1
  radps2rpm : Gain  Gain=convert.radps2rpm
  speed_rpm_to_workspace : ToWorkspace  VariableName=audit__mech__device_rpm  SampleTime=-1
  speed_to_workspace : ToWorkspace  VariableName=audit__mech__device_radps  SampleTime=-1
  torque_to_workspace : ToWorkspace  VariableName=audit__mech__device_Nm  SampleTime=-1
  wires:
  Mult/1 -> one half/1
  Square/1 -> Mult/1
  one half/1 -> KE_to_workspace/1
  radps2rpm/1 -> speed_rpm_to_workspace/1
  Mech Energy Nm radps/3 -> neg_energy_to_workspace/1
  Mech Energy Nm radps/2 -> pos_energy_to_workspace/1
  Mech Energy Nm radps/4 -> power_to_workspace/1
  Mech Energy Nm radps/1 -> energy_to_workspace/1
  iner_kgm2/1 -> inertia_to_workspace/1, Mult/2
  spd_radps/1 -> Mech Energy Nm radps/2, speed_to_workspace/1, radps2rpm/1, Square/1
  " trq_Nm"/1 -> Mech Energy Nm radps/1, torque_to_workspace/1

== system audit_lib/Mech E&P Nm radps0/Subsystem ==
  trq_Nm : Inport
  spd_radps : Inport  Port=2
  Enable : EnablePort  ZeroCross=off
  Mech Energy Nm radps : audit_lib/Mech Energy Nm radps
  energy_to_workspace : ToWorkspace  VariableName=audit__mech__device_kJ  SampleTime=-1
  neg_energy_to_workspace : ToWorkspace  VariableName=audit__mech__device_neg_kJ  SampleTime=-1
  pos_energy_to_workspace : ToWorkspace  VariableName=audit__mech__device_pos_kJ  SampleTime=-1
  power_to_workspace : ToWorkspace  VariableName=audit__mech__device_kW  SampleTime=-1
  radps2rpm : Gain  Gain=convert.radps2rpm
  speed_rpm_to_workspace : ToWorkspace  VariableName=audit__mech__device_rpm  SampleTime=-1
  speed_to_workspace : ToWorkspace  VariableName=audit__mech__device_radps  SampleTime=-1
  torque_to_workspace : ToWorkspace  VariableName=audit__mech__device_Nm  SampleTime=-1
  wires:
  Mech Energy Nm radps/1 -> energy_to_workspace/1
  Mech Energy Nm radps/4 -> power_to_workspace/1
  Mech Energy Nm radps/2 -> pos_energy_to_workspace/1
  Mech Energy Nm radps/3 -> neg_energy_to_workspace/1
  radps2rpm/1 -> speed_rpm_to_workspace/1
  trq_Nm/1 -> torque_to_workspace/1, Mech Energy Nm radps/1
  spd_radps/1 -> radps2rpm/1, speed_to_workspace/1, Mech Energy Nm radps/2

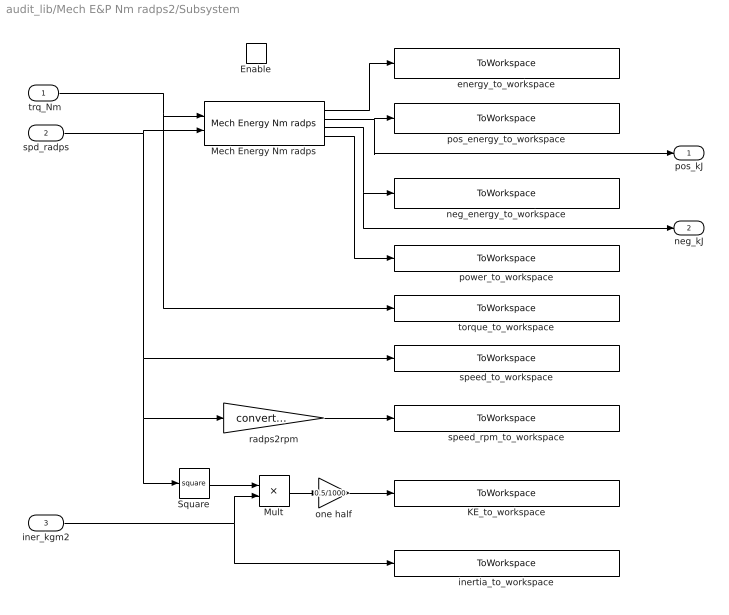
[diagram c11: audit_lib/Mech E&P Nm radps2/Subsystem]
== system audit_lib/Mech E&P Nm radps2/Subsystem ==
  " trq_Nm" : Inport
  spd_radps : Inport  Port=2
  iner_kgm2 : Inport  Port=3
  Enable : EnablePort  ZeroCross=off
  KE_to_workspace : ToWorkspace  VariableName=audit__mech__device_KE_kJ  SampleTime=-1
  Mech Energy Nm radps : audit_lib/Mech Energy Nm radps
  Mult : Product  Inputs=**
  Square : Math  Operator=square
  energy_to_workspace : ToWorkspace  VariableName=audit__mech__device_kJ  SampleTime=-1
  inertia_to_workspace : ToWorkspace  VariableName=audit__mech__device_kgm2  SampleTime=-1
  neg_energy_to_workspace : ToWorkspace  VariableName=audit__mech__device_neg_kJ  SampleTime=-1
  one half : Gain  Gain=0.5/1000
  pos_energy_to_workspace : ToWorkspace  VariableName=audit__mech__device_pos_kJ  SampleTime=-1
  power_to_workspace : ToWorkspace  VariableName=audit__mech__device_kW  SampleTime=-1
  radps2rpm : Gain  Gain=convert.radps2rpm
  speed_rpm_to_workspace : ToWorkspace  VariableName=audit__mech__device_rpm  SampleTime=-1
  speed_to_workspace : ToWorkspace  VariableName=audit__mech__device_radps  SampleTime=-1
  torque_to_workspace : ToWorkspace  VariableName=audit__mech__device_Nm  SampleTime=-1
  pos_kJ : Outport  InitialOutput=0
  neg_kJ : Outport  Port=2  InitialOutput=0
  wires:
  Mult/1 -> one half/1
  Square/1 -> Mult/1
  one half/1 -> KE_to_workspace/1
  radps2rpm/1 -> speed_rpm_to_workspace/1
  Mech Energy Nm radps/4 -> power_to_workspace/1
  Mech Energy Nm radps/1 -> energy_to_workspace/1
  iner_kgm2/1 -> inertia_to_workspace/1, Mult/2
  spd_radps/1 -> Mech Energy Nm radps/2, speed_to_workspace/1, radps2rpm/1, Square/1
  " trq_Nm"/1 -> Mech Energy Nm radps/1, torque_to_workspace/1
  Mech Energy Nm radps/2 -> pos_kJ/1, pos_energy_to_workspace/1
  Mech Energy Nm radps/3 -> neg_energy_to_workspace/1, neg_kJ/1

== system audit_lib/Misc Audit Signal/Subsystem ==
  In1 : Inport
  Enable : EnablePort
  To Workspace : ToWorkspace  VariableName=audit__mech__struct__var  SampleTime=-1
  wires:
  In1/1 -> To Workspace/1
